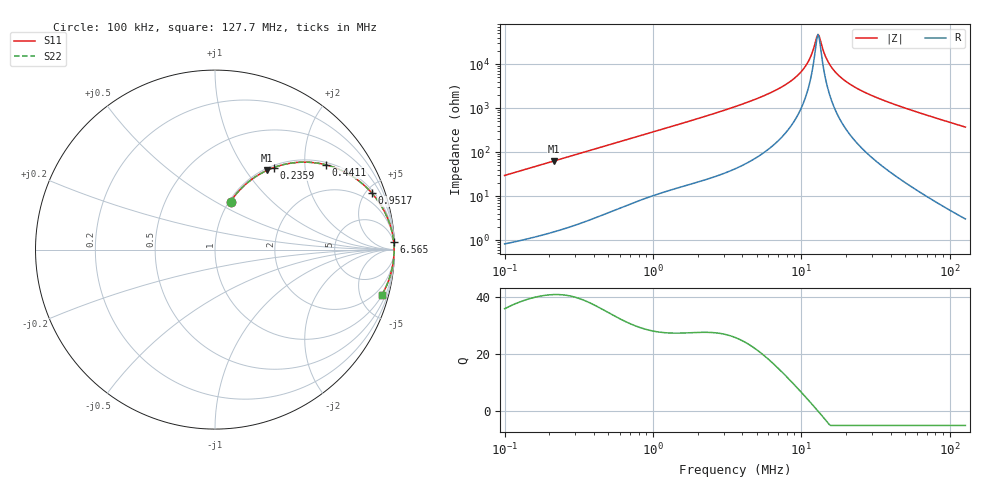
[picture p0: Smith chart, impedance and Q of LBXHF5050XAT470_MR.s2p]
! LBXHF5050XAT470_MR  S-PARAMETER MODEL  ( General Type )
! Model Generated by TAIYO YUDEN Corporation (http://www.ty-top.com)
! Version 1.0
! TAIYO YUDEN Control No. 201105NI43SB-FBB
! Copyright(c) 2020 TAIYO YUDEN CO.,LTD. All Rights Reserved.
! Product Description (link to TY-COMPAS)
! https://ds.yuden.co.jp/TYCOMPAS/or/detail?pn=LBXHF5050XAT470MMR&u=M
! Products Name : Inductors
! Characteristics :
!  Inductance : 47 uH , SRF(min) : 10 MHz , DC Resistance(max) : 0.36 Ohm
!  Rated Current : Saturation :850 mA , Temp Rise : 600 mA
!  Case Size : 5.0 x 5.0 / 0.197 x 0.197 [mm/inch] , Thickness : 3.1 / 0.122 [mm/inch]
!  (Conditions: Temperature = 25 degC , DC Bias Current/Voltage = 0A / 0V)
! External Node Assignments :
!  1  o---GGG---o  2
! GND o---------o GND
! Frequency Range : 0.1MHz  -  127.746476MHz  [ 402 STEP ]
# MHz S RI R 50
! Freq[MHz].  S11 Real  S11 Imag  S21 Real  S21 Imag  S12 Real  S12 Imag  S22 Real  S22 Imag
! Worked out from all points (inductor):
!   401 points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, 100 kHz to 127.7 MHz, reference 50 ohm
!   read as one part in series: L = 46.9 uH near 103.6 kHz
!   highest Q = 40.9 at 215.7 kHz (marker M1), where L = 46.7 uH
!   self-resonance near 12.95 MHz
!   S11 on the Smith chart (normalised r, x): 100 kHz: 1.02, +0.59; 235.9 kHz: 1.03, +1.38; 441.1 kHz: 1.07, +2.57; 951.7 kHz: 1.19, +5.48; 6.565 MHz: 4, +49; 127.7 MHz: 1.06, -7.41
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0.1  0.0865 0.2675  0.9135 -0.2675  0.9135 -0.2675  0.0865 0.2675
0.215741  0.2906 0.442  0.7094 -0.442  0.7094 -0.442  0.2906 0.442
0.235918  0.3275 0.4572  0.6725 -0.4572  0.6725 -0.4572  0.3275 0.4572
0.33137  0.4844 0.4872  0.5156 -0.4872  0.5156 -0.4872  0.4844 0.4872
0.441131  0.6198 0.4718  0.3802 -0.4718  0.3802 -0.4718  0.6198 0.4718
0.9517  0.8741 0.3146  0.1259 -0.3146  0.1259 -0.3146  0.8741 0.3146
1.098062  0.9005 0.2819  0.0995 -0.2819  0.0995 -0.2819  0.9005 0.2819
3.574164  0.988 0.0912  0.012 -0.0912  0.012 -0.0912  0.988 0.0912
6.564688  0.9959 0.0405  0.00413 -0.0405  0.00413 -0.0405  0.9959 0.0405
8.135881  0.997 0.0267  0.00302 -0.0267  0.00302 -0.0267  0.997 0.0267
9.556469  0.9975 0.0172  0.00252 -0.0172  0.00252 -0.0172  0.9975 0.0172
10.83075  0.9977 0.0101  0.00227 -0.0101  0.00227 -0.0101  0.9977 0.0101
11.84371  0.9978 0.00509  0.00216 -0.00509  0.00216 -0.00509  0.9978 0.00509
12.72188  0.9979 0.00113  0.00212 -0.00113  0.00212 -0.00113  0.9979 0.00113
13.18509  0.9979 -0.000841  0.00211 0.000841  0.00211 0.000841  0.9979 -0.000841
14.41825  0.9979 -0.00578  0.00212 0.00578  0.00212 0.00578  0.9979 -0.00578
15.21283  0.9978 -0.00877  0.00215 0.00877  0.00215 0.00877  0.9978 -0.00877
16.34081  0.9978 -0.0128  0.00223 0.0128  0.00223 0.0128  0.9978 -0.0128
18.19151  0.9976 -0.019  0.00241 0.019  0.00241 0.019  0.9976 -0.019
24.65407  0.9965 -0.0378  0.00346 0.0378  0.00346 0.0378  0.9965 -0.0378
39.24654  0.9925 -0.0739  0.00751 0.0739  0.00751 0.0739  0.9925 -0.0739
127.7465  0.9304 -0.2505  0.0696 0.2505  0.0696 0.2505  0.9304 -0.2505
